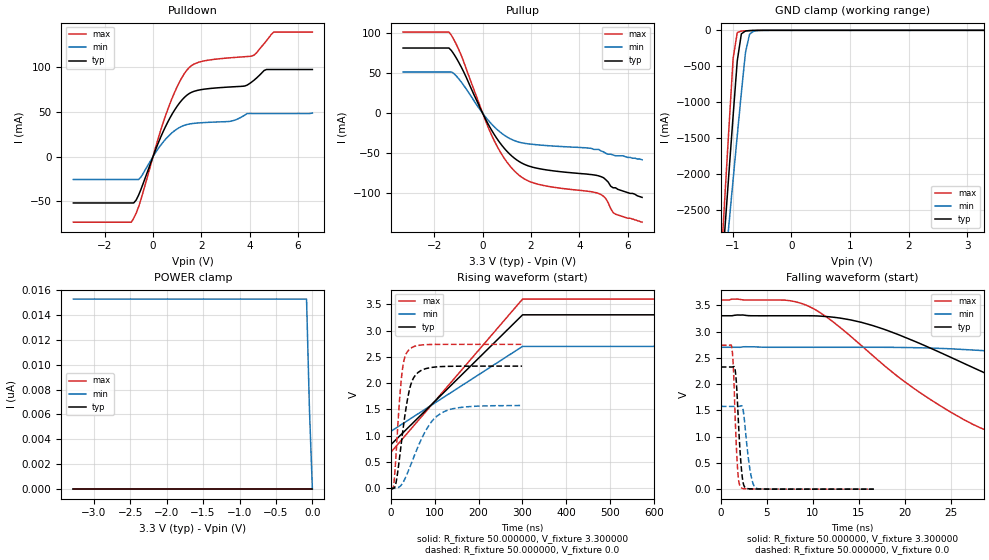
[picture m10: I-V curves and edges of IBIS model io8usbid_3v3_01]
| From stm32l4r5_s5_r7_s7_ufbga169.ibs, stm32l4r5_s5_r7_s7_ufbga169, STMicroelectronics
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|   Model io8usbid_3v3_01
[Model]  io8usbid_3v3_01
Model_type I/O
Polarity   Non-Inverting
Enable   Active-Low
Vinl =   0.990000V
Vinh =   2.310000V
Vmeas =  1.650000V
Cref =   100.000000nF
Rref =   1.000000k
Vref =   3.300000V
C_comp   2.116400pF   2.092700pF   2.152900pF
[Temperature Range]   25.000000   0.125000k   -40.000000
[Pullup Reference]   3.300000V   2.700000V   3.600000V
[Pulldown Reference]   0.0V   0.0V   0.0V
[POWER Clamp Reference]   3.300000V   2.700000V   3.600000V
[GND Clamp Reference]   0.0V   0.0V   0.0V
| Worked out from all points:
|   slope of the pulldown table from 0 to 0.495 V, typ, clamps not added: 15.4 ohm
|   slope of the pullup table from 0 to 0.495 V, typ, clamps not added: 18.1 ohm
|   GND clamp passes 1 mA (typ) near -0.59 V on its own axis
|   rising waveform, R_fixture 50.000000, V_fixture 3.300000: 20-80 % time 180ns typ, 180ns min, 180ns max; typ from 0.835 V to 3.3 V
|   rising waveform, R_fixture 50.000000, V_fixture 0.0: 20-80 % time 23.9ns typ, 53.2ns min, 14.3ns max; typ from 0 V to 2.33 V
|   falling waveform, R_fixture 50.000000, V_fixture 3.300000: 20-80 % time 21ns typ, 41.6ns min, 13.6ns max; typ from 3.3 V to 0.835 V
|   falling waveform, R_fixture 50.000000, V_fixture 0.0: 20-80 % time 450ps typ, 628ps min, 372ps max; typ from 2.33 V to 0 V
[Pulldown]
|Voltage   I(typ)   I(min)   I(max)
-3.3V     -51.62mA   -25.53mA   -73.04mA
-900mV    -51.62mA   -25.53mA   -73.04mA
-500mV    -36.51mA   -22.79mA   -47.71mA
200mV     14.03mA    8.316mA    18.9mA
700mV     42.99mA    24.4mA     58.9mA
1.2V      63.06mA    33.8mA     88.14mA
1.6V      71.64mA    36.67mA    101.4mA
3.2V      77.51mA    39.29mA    110mA
4.1V      83.27mA    47.98mA    111.9mA
4.6V      95.83mA    47.98mA    125.7mA
5V        96.94mA    47.98mA    138.6mA
6.6V      96.94mA    48.43mA    138.6mA
[Pullup]
|Voltage   I(typ)   I(min)   I(max)
-3.3V     81.68mA    51.74mA    101.6mA
-1.4V     81.68mA    51.74mA    101.6mA
-900mV    58.51mA    39.6mA     73.28mA
100mV     -6.165mA   -3.962mA   -8.038mA
500mV     -27.53mA   -17.49mA   -35.6mA
1V        -47.29mA   -29.38mA   -60.81mA
1.5V      -60.05mA   -35.95mA   -77.15mA
2.4V      -69.45mA   -39.66mA   -89.34mA
4.8V      -78.1mA    -45mA      -100.1mA
5.1V      -83mA      -50mA      -106.7mA
5.5V      -93mA      -53mA      -126mA
6.6V      -105mA     -58mA      -136mA
[GND_clamp]
|Voltage   I(typ)   I(min)   I(max)
-3.3V     -9.914A    -9.595A    -9.188A
-1.2V     -3.541A    -3.911A    -3.279A
-1.13V    -2.75A     -3.295A    -2.301A
-1.06V    -1.963A    -2.68A     -1.33A
-990mV    -1.183A    -2.069A    -386.7mA
-920mV    -424.7mA   -1.463A    -31.42mA
-850mV    -49.12mA   -868.7mA   -10.48mA
-780mV    -9.121mA   -308.3mA   -6.715mA
-710mV    -3.648mA   -53.81mA   -3.986mA
-640mV    -1.726mA   -11.03mA   -1.885mA
-430mV    -22.46uA   -116.8uA   -9.748uA
3.28V     0A         0A         0A
[POWER_clamp]
|Voltage   I(typ)   I(min)   I(max)
-3.28V    0A         15.27nA    0A
-80mV     0A         15.27nA    0A
-40mV     0A         6.354nA    0A
0V        0A         0A         0A
[Ramp]
| variable   typ   min   max
dV/dt_r  1.39476/23.89676n   0.94506/53.25050n   1.64316/14.30463n
dV/dt_f  1.47899/21.07093n   0.96780/44.63517n   1.74604/13.57871n
R_load = 50.000000
[Rising Waveform]
R_fixture= 50.000000
V_fixture= 3.300000
V_fixture_min= 2.700000
V_fixture_max= 3.600000
|time   V(typ)   V(min)   V(max)
0s        835mV      1.087V     689.9mV
300.3ns   3.3V       2.7V       3.6V
600.6ns   3.3V       2.7V       3.6V
29.73us   3.3V       2.7V       3.6V
[Rising Waveform]
R_fixture= 50.000000
V_fixture= 0.0
V_fixture_min= 0.0
V_fixture_max= 0.0
|time   V(typ)   V(min)   V(max)
0s        3.26nV     60.03nV    3.11nV
6.607ns   3.522mV    -135.5uV   106.8mV
13.21ns   202.3mV    4.86mV     910.9mV
19.82ns   617.9mV    33.43mV    1.739V
25.83ns   1.032V     93.35mV    2.261V
31.23ns   1.371V     175.8mV    2.492V
41.44ns   1.859V     373.8mV    2.64V
61.86ns   2.206V     799.7mV    2.718V
112.3ns   2.315V     1.419V     2.738V
299.1ns   2.325V     1.575V     2.739V
[Falling Waveform]
R_fixture= 50.000000
V_fixture= 3.300000
V_fixture_min= 2.700000
V_fixture_max= 3.600000
|time   V(typ)   V(min)   V(max)
0s        3.3V       2.7V       3.6V
9.61ns    3.3V       2.7V       3.476V
16.52ns   3.113V     2.7V       2.541V
24.92ns   2.513V     2.672V     1.471V
29.73ns   2.129V     2.619V     1.061V
34.53ns   1.78V      2.543V     888.3mV
45.35ns   1.198V     2.309V     774.6mV
57.66ns   992.8mV    1.996V     728.6mV
92.79ns   866.9mV    1.304V     696mV
149.5ns   835mV      1.087V     689.9mV
[Falling Waveform]
R_fixture= 50.000000
V_fixture= 0.0
V_fixture_min= 0.0
V_fixture_max= 0.0
|time   V(typ)   V(min)   V(max)
0s        2.325V     1.575V     2.739V
1.201ns   2.324V     1.575V     2.691V
1.368ns   2.331V     1.575V     2.301V
1.535ns   2.294V     1.575V     1.489V
1.802ns   1.677V     1.575V     442.9mV
2.202ns   455.9mV    1.587V     29.18mV
2.569ns   48.02mV    1.304V     8.052mV
3.203ns   5.591mV    333.7mV    4.377mV
3.804ns   3.091mV    21.86mV    3.334mV
16.62ns   3.26nV     60.03nV    3.11nV
